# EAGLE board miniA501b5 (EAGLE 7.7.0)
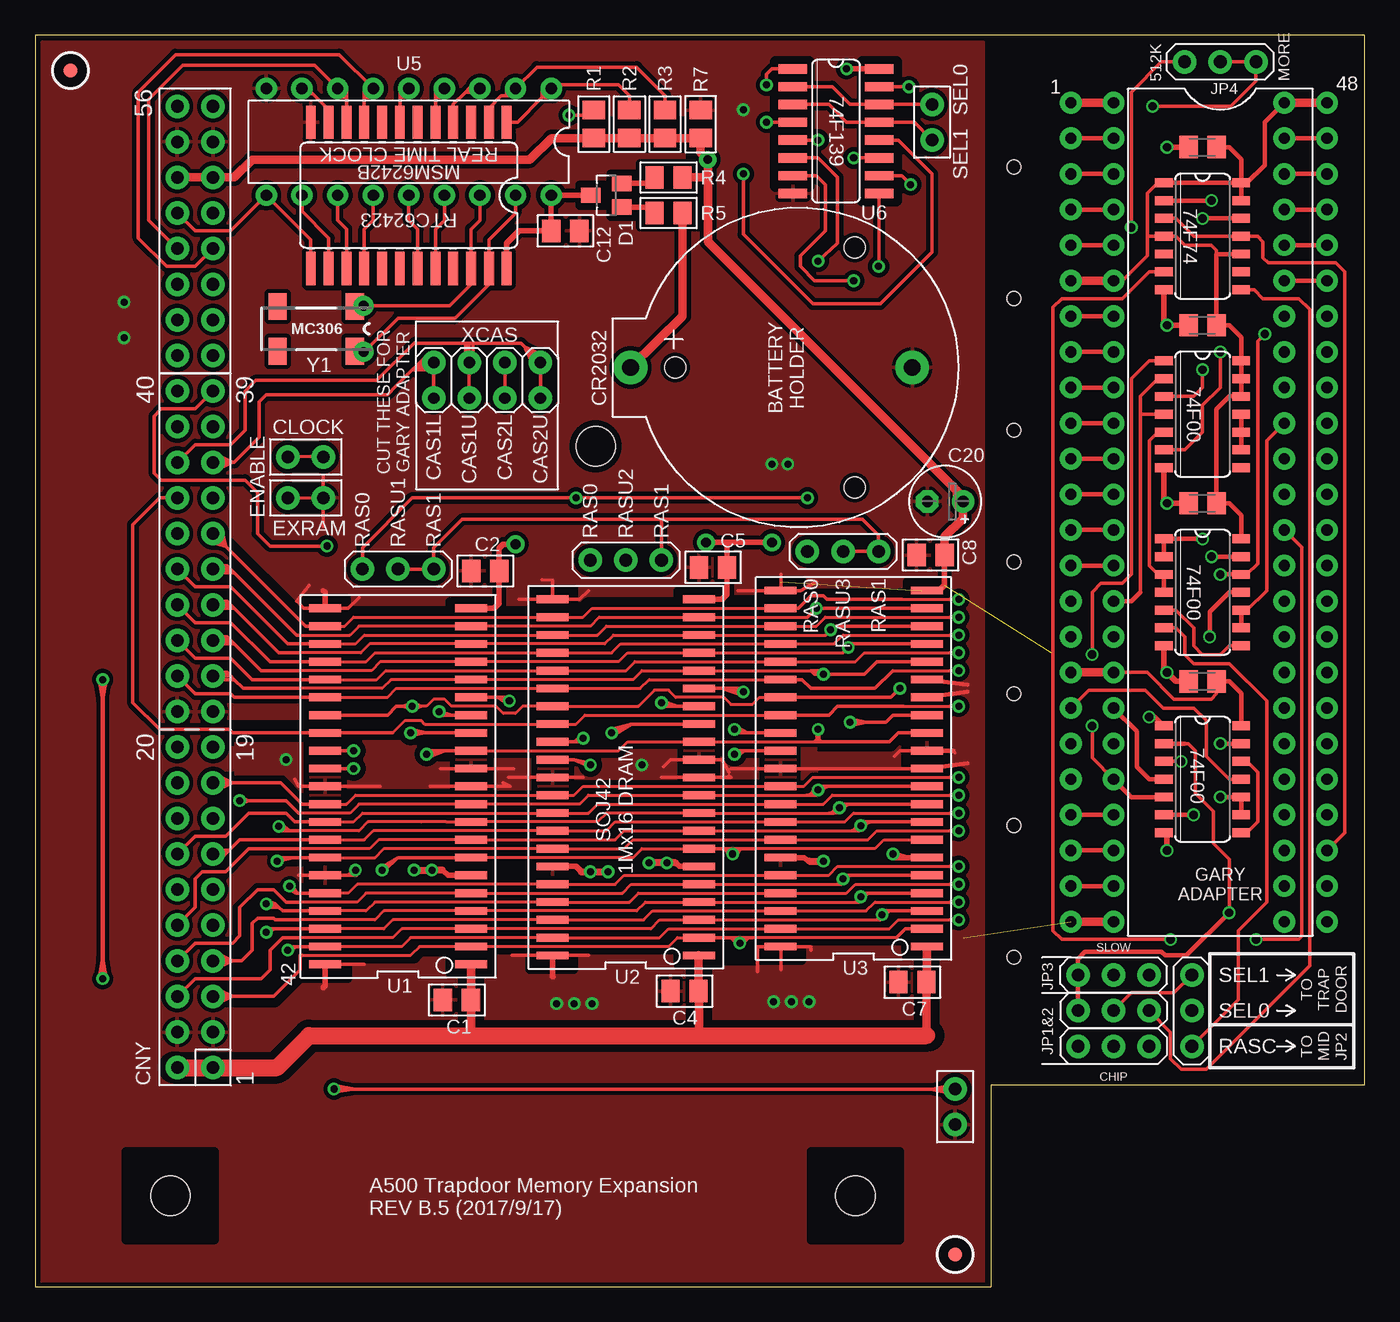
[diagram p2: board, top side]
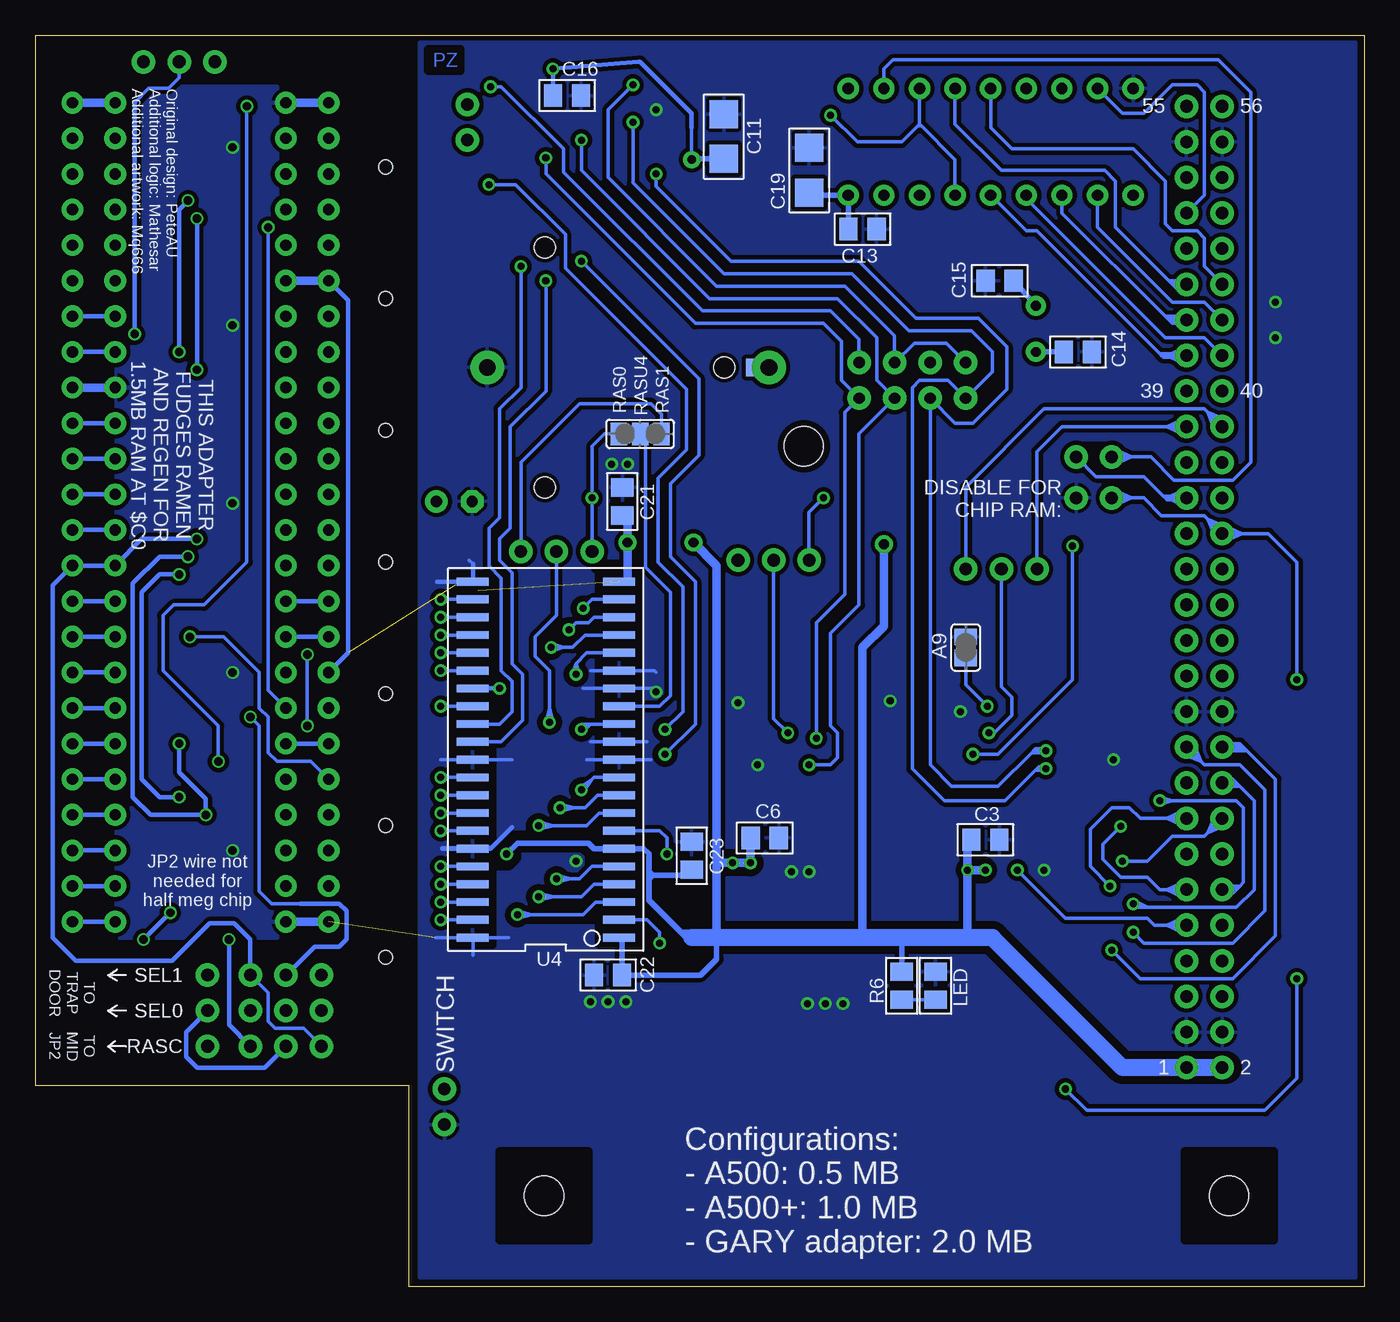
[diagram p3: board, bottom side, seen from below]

Size 94.87 x 89.28 mm. Coordinates in mm from the lower left corner, seen from the top.
Outline: 0,0 68.2,0 68.2,14.35 94.87,14.35 94.87,89.28 0,89.28 0,0
Copper layers (1*16): Top 0.035mm / dielectric 1.5mm / Bottom 0.035mm
Design rules "SeeedStudio_DRU_no_angle_2layer *": minimum track width 6mil, minimum drill 12mil, track to track 10mil, track to pad 10mil, pad to pad 10mil, via to via 10mil, smd to smd 0mil, copper to edge 10mil, drill to drill 10mil, minimum pad ring 10mil, minimum via ring 6mil, stop-mask expansion 2mil, vias tented up to drill 25mil, thermal gap 10mil
Holes 2.8 mm at 9.65,6.48 58.55,6.48 40.01,59.94
Holes 1 mm at 69.85,51.69 69.85,32.89 69.85,70.48 69.85,79.88 69.85,42.29 69.85,23.49 69.85,61.09
tRestrict: area 19.2,22 to 22.4,23.5; area 19.2,47.6 to 22.2,49.1; area 45.8,34.7 to 46,43.2; area 45.8,35.3 to 46,38.1; area 38.4,34.7 to 38.5,38; area 22.1,34.9 to 22.2,36.7; area 35.4,47.4 to 38.5,49.8; area 32.6,41.1 to 34.7,42.4; area 27.9,40.4 to 29.7,41.7; area 38.4,28.8 to 42.9,30.4; area 54.6,28.6 to 58.3,31.2; area 48.9,41.9 to 50.9,43.2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; 65 lines
bRestrict: area 64.5,86.7 to 66.8,88.3; area 6.5,3.3 to 12.8,9.7; area 55.4,3.3 to 61.7,9.7; area 52.8,42.8 to 53.6,43.8; area 52.8,37.7 to 53.6,38.7; area 62.2,49.9 to 65.2,50.8; area 51.8,50.7 to 54.5,50.8; area 62.2,24.4 to 64.8,24.5; area 55.4,39.3 to 56.3,40.2; area 55.8,43.2 to 56.7,44.1; area 55.3,47.9 to 56.2,48.8; area 56.3,46.4 to 57.2,47.3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; 15 lines

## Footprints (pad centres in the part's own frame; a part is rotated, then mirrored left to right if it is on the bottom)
SJ = smd 1.168 x 1.6: 1 -0.762,0; 2 0.762,0
CR2032-THRU = drill 1.2 pad 2.4: + 0,-11.1; - 0,9 | smd 1.27 x 0.635 bottom: +2 0,-9.763 | hole 1.5: 8.55,4.9; 0,-7.9; -8.55,4.9
C0805KPZ = smd 1.3 x 1.6: P$1 -1,0; P$2 1,0
C0805K = smd 1.3 x 1.6: 1 -1,0; 2 1,0
C1206PZ = smd 2 x 2.05: P$1 -1.6,0; P$2 1.6,0
E2,5-5 = drill 0.813 pad 1.6: + -1.27,0 | drill 0.813 pad 1.6 octagon: - 1.27,0
1X02 = drill 0.9 pad 1.676: 1 -1.27,0; 2 1.27,0
2X20 = drill 0.9 pad 1.676: 1 -24.13,-1.27; 2 -24.13,1.27; 3 -21.59,-1.27; 4 -21.59,1.27; 5 -19.05,-1.27; 6 -19.05,1.27; 7 -16.51,-1.27; 8 -16.51,1.27; 9 -13.97,-1.27; 10 -13.97,1.27; 11 -11.43,-1.27; 12 -11.43,1.27; 13 -8.89,-1.27; 14 -8.89,1.27; 15 -6.35,-1.27; 16 -6.35,1.27; 17 -3.81,-1.27; 18 -3.81,1.27; 19 -1.27,-1.27; 20 -1.27,1.27; 21 1.27,-1.27; 22 1.27,1.27; 23 3.81,-1.27; 24 3.81,1.27; 25 6.35,-1.27; 26 6.35,1.27; 27 8.89,-1.27; 28 8.89,1.27; 29 11.43,-1.27; 30 11.43,1.27; 31 13.97,-1.27; 32 13.97,1.27; 33 16.51,-1.27; 34 16.51,1.27; 35 19.05,-1.27; 36 19.05,1.27; 37 21.59,-1.27; 38 21.59,1.27; 39 24.13,-1.27; 40 24.13,1.27
2X08 = drill 0.9 pad 1.676: 1 -8.89,-1.27; 2 -8.89,1.27; 3 -6.35,-1.27; 4 -6.35,1.27; 5 -3.81,-1.27; 6 -3.81,1.27; 7 -1.27,-1.27; 8 -1.27,1.27; 9 1.27,-1.27; 10 1.27,1.27; 11 3.81,-1.27; 12 3.81,1.27; 13 6.35,-1.27; 14 6.35,1.27; 15 8.89,-1.27; 16 8.89,1.27
SOT23 = smd 1.1 x 1.4: 1 -0.85,-1.1; 2 0.85,-1.1; 3 0,1.1
DIL48 = drill 0.8 pad 1.55: 1 -29.21,-7.62; 2 -26.67,-7.62; 3 -24.13,-7.62; 4 -21.59,-7.62; 5 -19.05,-7.62; 6 -16.51,-7.62; 7 -13.97,-7.62; 8 -11.43,-7.62; 9 -8.89,-7.62; 10 -6.35,-7.62; 11 -3.81,-7.62; 12 -1.27,-7.62; 13 1.27,-7.62; 14 3.81,-7.62; 15 6.35,-7.62; 16 8.89,-7.62; 17 11.43,-7.62; 18 13.97,-7.62; 19 16.51,-7.62; 20 19.05,-7.62; 21 21.59,-7.62; 22 24.13,-7.62; 23 26.67,-7.62; 24 29.21,-7.62; 25 29.21,7.62; 26 26.67,7.62; 27 24.13,7.62; 28 21.59,7.62; 29 19.05,7.62; 30 16.51,7.62; 31 13.97,7.62; 32 11.43,7.62; 33 8.89,7.62; 34 6.35,7.62; 35 3.81,7.62; 36 1.27,7.62; 37 -1.27,7.62; 38 -3.81,7.62; 39 -6.35,7.62; 40 -8.89,7.62; 41 -11.43,7.62; 42 -13.97,7.62; 43 -16.51,7.62; 44 -19.05,7.62; 45 -21.59,7.62; 46 -24.13,7.62; 47 -26.67,7.62; 48 -29.21,7.62
SO14 = smd 0.635 x 1.27: 1 -3.81,-2.756; 2 -2.54,-2.756; 3 -1.27,-2.756; 4 0,-2.756; 5 1.27,-2.756; 6 2.54,-2.756; 7 3.81,-2.756; 8 3.81,2.756; 9 2.54,2.756; 10 1.27,2.756; 11 0,2.756; 12 -1.27,2.756; 13 -2.54,2.756; 14 -3.81,2.756
1X03 = drill 0.9 pad 1.676: 1 -2.54,0; 2 0,0; 3 2.54,0
1X01 = drill 0.7 pad 1.422: 1 0,0
2X04 = drill 0.813 pad 1.676: 1 -3.81,-1.27; 2 -3.81,1.27; 3 -1.27,-1.27; 4 -1.27,1.27; 5 1.27,-1.27; 6 1.27,1.27; 7 3.81,-1.27; 8 3.81,1.27
M0805PZ = smd 1.3 x 1.6: P$1 -1,0; P$2 1,0
SJ_2 = smd 1.168 x 1.6: 1 -1.524,0; 2 0,0; 3 1.524,0
SOJ40 = smd 0.559 x 2.286: 1 -10.16,-5.22; 2 -8.89,-5.22; 3 -7.62,-5.22; 4 -6.35,-5.22; 5 -5.08,-5.22; 6 -3.81,-5.22; 7 -2.54,-5.22; 8 -1.27,-5.22; 9 0,-5.22; 10 1.27,-5.22; 11 2.54,-5.22; 12 3.81,-5.22; 13 5.08,-5.22; 14 6.35,-5.22; 15 7.62,-5.22; 16 8.89,-5.22; 17 10.16,-5.22; 18 11.43,-5.22; 19 12.7,-5.22; 20 13.97,-5.22; 21 15.24,-5.22; 22 15.24,5.22; 23 13.97,5.22; 24 12.7,5.22; 25 11.43,5.22; 26 10.16,5.22; 27 8.89,5.22; 28 7.62,5.22; 29 6.35,5.22; 30 5.08,5.22; 31 3.81,5.22; 32 2.54,5.22; 33 1.27,5.22; 34 0,5.22; 35 -1.27,5.22; 36 -2.54,5.22; 37 -3.81,5.22; 38 -5.08,5.22; 39 -6.35,5.22; 40 -7.62,5.22; 41 -8.89,5.22; 42 -10.16,5.22
DIL18 = drill 0.813 pad 1.524: 1 -10.16,-3.81; 2 -7.62,-3.81; 3 -5.08,-3.81; 4 -2.54,-3.81; 5 0,-3.81; 6 2.54,-3.81; 7 5.08,-3.81; 8 7.62,-3.81; 9 10.16,-3.81; 10 10.16,3.81; 11 7.62,3.81; 12 5.08,3.81; 13 2.54,3.81; 14 0,3.81; 15 -2.54,3.81; 16 -5.08,3.81; 17 -7.62,3.81; 18 -10.16,3.81
SO16 = smd 0.66 x 2.032: 1 -4.445,-3.073; 2 -3.175,-3.073; 3 -1.905,-3.073; 4 -0.635,-3.073; 5 0.635,-3.073; 6 1.905,-3.073; 7 3.175,-3.073; 8 4.445,-3.073; 9 4.445,3.073; 10 3.175,3.073; 11 1.905,3.073; 12 0.635,3.073; 13 -0.635,3.073; 14 -1.905,3.073; 15 -3.175,3.073; 16 -4.445,3.073
SOP24 = smd 0.711 x 2.362: 1 -6.985,-5.22; 2 -5.715,-5.22; 3 -4.445,-5.22; 4 -3.175,-5.22; 5 -1.905,-5.22; 6 -0.635,-5.22; 7 0.635,-5.22; 8 1.905,-5.22; 9 3.175,-5.22; 10 4.445,-5.22; 11 5.715,-5.22; 12 6.985,-5.22; 13 6.985,5.22; 14 5.715,5.22; 15 4.445,5.22; 16 3.175,5.22; 17 1.905,5.22; 18 0.635,5.22; 19 -0.635,5.22; 20 -1.905,5.22; 21 -3.175,5.22; 22 -4.445,5.22; 23 -5.715,5.22; 24 -6.985,5.22
FIDUCIAL_1MM = smd 1 x 1: 1 0,0
MC-306 = smd 1.3 x 1.9: 1 -2.75,-1.6; 2 2.75,-1.6; 3 2.75,1.6; 4 -2.75,1.6

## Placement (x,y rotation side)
A9  [SJ]  28.45,45.59 270 bottom
BAT1  [CR2032-THRU]  53.59,65.57 270 top
C1  100nF  [C0805KPZ]  30.1,20.45 0 top
C2  100nF  [C0805KPZ]  32.13,51.05 0 top
C3  100nF  [C0805KPZ]  27.05,31.88 180 bottom
C4  100nF  [C0805KPZ]  46.35,21.08 0 top
C5  100nF  [C0805KPZ]  48.39,51.31 0 top
C6  100nF  [C0805KPZ]  42.8,32 180 bottom
C7  100nF  [C0805KPZ]  62.61,21.72 0 top
C8  100nF  [C0805KPZ]  63.91,52.19 0 top
C9  100n  [C0805K]  83.31,43.18 180 top
C11  TANT  [C1206PZ]  45.72,82.04 90 bottom
C12  100nF  [C0805KPZ]  37.85,75.31 180 top
C13  4.7uF 10V  [C0805KPZ]  35.81,75.44 0 bottom
C14  22pF  [C0805KPZ]  20.45,66.67 0 bottom
C15  22pF  [C0805KPZ]  26.04,71.75 180 bottom
C16  100nF  [C0805KPZ]  56.9,84.96 0 bottom
C17  100n  [C0805K]  83.31,55.88 180 top
C18  100n  [C0805K]  83.31,68.58 180 top
C19  [C1206PZ]  39.62,79.63 90 bottom
C20  [E2,5-5]  64.95,56.01 180 top
C21  100nF  [C0805KPZ]  52.96,56.01 270 bottom
C22  100nF  [C0805KPZ]  53.98,22.23 0 bottom
C23  100nF  [C0805KPZ]  48.01,30.73 270 bottom
C24  100n  [C0805K]  83.31,81.28 180 top
CLOCK  [1X02]  19.3,59.18 0 top
CNY  [2X20]  11.43,39.75 90 top
CNY2  [2X08]  11.43,75.31 90 top
D1  BAT721C  [SOT23]  40.77,77.85 90 top
EXRAM  [1X02]  19.3,56.26 0 top
GARY  [DIL48]  84.58,55.24 270 top
IC1  74F00  [SO14]  83.31,36.2 270 top
IC2  74F00  [SO14]  83.31,49.53 270 top
IC3  74F00  [SO14]  83.31,62.23 270 top
IC4  74F74  [SO14]  83.31,74.93 270 top
J8  [1X03]  82.55,19.68 90 top
JP1  [1X03]  25.91,51.18 0 top
JP2  [1X03]  76.96,17.14 0 top
JP3  [1X01]  23.44,66.67 0 top
JP4  [1X01]  23.44,69.98 0 top
JP5  [1X03]  57.66,52.45 0 top
JP6  [1X03]  76.96,19.68 0 top
JP7  [1X03]  42.16,51.82 0 top
JP8  [1X03]  76.96,22.23 180 top
JP9  [1X03]  84.58,87.38 180 top
JP10  [2X04]  32.26,64.64 180 top
LED  LED  [M0805PZ]  30.61,21.46 270 bottom
R1  10K  [M0805PZ]  39.88,82.93 270 top
R2  10K  [M0805PZ]  42.42,82.93 270 top
R3  10K  [M0805PZ]  44.96,82.93 270 top
R4  470  [M0805PZ]  45.21,79.12 0 top
R5  470  [M0805PZ]  45.21,76.58 0 top
R6  1K  [M0805PZ]  33.02,21.46 90 bottom
R7  100K  [C0805KPZ]  47.5,82.93 90 top
SEL[0_1]  [1X02]  64.01,83.06 270 top
SJ1  [SJ_2]  51.69,60.83 0 bottom
SOCKET(MOBO)  [DIL48]  81.53,55.24 270 top
SWITCH  [1X02]  65.66,12.83 270 top
U1  [SOJ40]  25.91,33.15 90 top
U2  [SOJ40]  42.16,33.78 90 top
U3  [SOJ40]  58.42,34.42 90 top
U4  [SOJ40]  58.42,35.05 90 bottom
U5  OKI MSM6242B  [DIL18]  26.67,81.66 180 top
U6  74F139D  [SO16]  57.15,82.42 270 top
U55  RTC72421SOP24  [SOP24]  26.67,77.85 180 top
U$1  FIDUCIAL  [FIDUCIAL_1MM]  2.54,86.74 0 top
U$2  FIDUCIAL  [FIDUCIAL_1MM]  65.66,2.29 0 top
Y1  MC-306  [MC-306]  20.07,68.33 180 top

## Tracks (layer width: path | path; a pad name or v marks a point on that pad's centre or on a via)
/A19
  Top 0.254: 80.14,50.8 79.5,51.43 79.5,60.32 80.14,60.96
  Top 0.305: IC2.4 IC2.3 80.14,50.8 | 80.14,60.96 IC3.5
/A19_FF  (via drill 0.6)
  Top 0.254: v81.03,24.77 73.28,24.77 72.64,25.4 72.64,69.85 73.28,70.48 77.6,70.48 79.5,72.39 IC4.6
  Bottom 0.305: JP2.3 81.03,18.67 v81.03,24.77
/BLIT
  Top 0.254: 78.87,49.53 78.87,62.23 | 78.87,62.23 78.87,63.5 80.14,64.77 | IC3.4 78.87,62.23
  Top 0.305: GARY.15 78.23,48.89 78.87,49.53 | 80.14,64.77 IC3.2
  Bottom 0.305: SOCKET(MOBO).15 GARY.15
/GARY_RAMEN  (via drill 0.6)
  Top 0.254: GARY.20 75.44,37.72 v75.44,40 | v75.44,45.09 75.44,49.53 76.07,50.16 77.6,50.16 78.23,50.8 78.23,64.77 79.5,66.04 IC3.1
  Top 0.305: IC1.5 78.23,34.92 GARY.20
  Bottom 0.254: v75.44,40 v75.44,45.09
/GARY_RAMEN_FF
  Top 0.254: IC4.8 87,71.12 87.63,70.48 90.2,70.48 90.96,69.72 90.96,22.88 83.57,15.49 81.79,15.49 81.03,16.26 81.03,18.16 JP6.3
/GARY_REGEN  (via drill 0.6)
  Top 0.254: v78.23,75.56 78.23,85.22 80.39,87.38 JP9.3
  Top 0.305: IC1.4 79.5,36.2 78.61,37.08 78.61,39.62 GARY.18
  Bottom 0.254: GARY.18 78.23,42.54 v78.23,75.56
/NEW_RAMEN  (via drill 0.6)
  Top 0.305: IC2.11 85.22,49.53 83.82,48.13 v83.82,46.35
  Bottom 0.254: SOCKET(MOBO).20 75.18,37.46 77.6,37.46 78.23,38.1 78.23,40.64 78.87,41.27 78.87,43.81 81.41,46.35 v83.82,46.35
/NEW_REGEN
  Top 0.254: IC1.11 85.22,36.2 83.57,37.85 83.57,40.39 82.68,41.27 80.52,41.27 79.25,42.54 75.18,42.54 SOCKET(MOBO).18
A0  (via drill 0.5 pad 0.9)
  Top 0.203: 18.8,42.67 24.77,42.67 25.4,43.31 U1.17 42.67,43.31 43.31,43.94 U2.17 55.37,43.94
  Top 0.254: U3.17 60.07,44.58 59.18,43.69 v56.26,43.69 55.63,43.69 55.37,43.94 56.26,43.94 | CNY.23 13.97,43.56 | 13.97,43.56 14.22,43.31 | 14.22,43.31 14.86,42.67 18.8,42.67 | 14.22,43.31 12.7,43.31 | 13.97,43.56 13.72,43.81 12.7,43.81
  Bottom 0.254: U4.17 55.5,45.21 56.26,44.45 | 56.26,44.45 v56.26,43.69 | 56.26,44.45 56.01,43.69 | 56.26,44.45 56.52,43.69
A1  (via drill 0.5 pad 0.9)
  Top 0.203: 18.8,43.94 24,43.94 24.64,44.58 U1.18 41.66,44.58 42.29,45.21 U2.18 57.66,45.21
  Top 0.254: 18.8,43.94 16.13,43.94 14.22,45.85 | 57.66,45.21 v58.04,45.59 58.29,45.85 U3.18 | 14.22,45.85 13.97,46.1 | 13.97,46.1 CNY.25 | 14.22,45.85 12.7,45.85 | 13.97,46.1 13.72,46.35 12.7,46.35
  Bottom 0.254: U4.18 55.63,46.48 56.52,45.59 57.15,45.59 | 57.15,45.59 v58.04,45.59 | 57.15,45.59 58.04,45.85 | 57.15,45.59 58.04,45.34
A2  (via drill 0.5 pad 0.9)
  Top 0.203: 18.8,45.21 23.24,45.21 23.88,45.85 U1.19 40.64,45.85 41.27,46.48 U2.19 56.39,46.48
  Top 0.254: 18.8,45.21 17.4,45.21 14.22,48.39 | 56.39,46.48 v56.77,46.86 57.02,47.12 U3.19 | CNY.27 13.97,48.64 | 13.97,48.64 14.22,48.39 | 14.22,48.39 12.7,48.39 | 13.97,48.64 13.72,48.89 12.7,48.89
  Bottom 0.254: U4.19 54.99,47.75 55.37,47.37 56.26,47.37 v56.77,46.86
A3  (via drill 0.5 pad 0.9)
  Top 0.203: 55.12,47.75 U2.20 40.26,47.75 39.62,47.12 U1.20 23.11,47.12 22.48,46.48 18.8,46.48
  Top 0.254: 55.12,47.75 v55.75,48.39 U3.20 | 18.8,46.48 18.67,46.48 14.22,50.93 | CNY.29 13.97,51.18 | 13.97,51.18 14.22,50.93 | 14.22,50.93 12.7,50.93 | 13.97,51.18 13.72,51.43 12.7,51.43
  Bottom 0.254: U4.20 55.12,49.02 v55.75,48.39
A4  (via drill 0.5 pad 0.9)
  Top 0.203: U1.23 22.1,47.12 22.73,47.75 U2.23 39.12,47.75 39.75,48.39 U3.23 | 61.85,49.02 65.28,49.02
  Top 0.254: U1.23 19.3,47.12 13.59,52.83 | U3.23 54.48,48.39 55.37,49.28 56.26,49.28 56.52,49.02 61.85,49.02 | 65.28,49.02 v65.91,49.02 | CNY.31 13.59,52.83 | 13.59,52.83 12.57,53.09 | 13.59,52.83 13.34,53.97
  Bottom 0.254: v65.91,49.02 U4.23
A5  (via drill 0.5 pad 0.9)
  Top 0.203: U1.24 22.86,45.85 23.49,46.48 U2.24 | 36.96,46.48 U2.24 | U2.24 40.13,46.48 40.77,47.12 U3.24 55.75,47.12 56.39,47.75 65.28,47.75
  Top 0.254: U1.24 18.03,45.85 13.97,49.91 11.43,49.91 CNY.30 | 65.28,47.75 v65.91,47.75
  Bottom 0.254: v65.91,47.75 U4.24
A6  (via drill 0.5 pad 0.9)
  Top 0.203: U1.25 23.62,44.58 24.26,45.21 U2.25 | 36.96,45.21 U2.25 | U2.25 41.15,45.21 41.78,45.85 U3.25 57.02,45.85 57.66,46.48 65.28,46.48
  Top 0.254: U1.25 16.76,44.58 13.97,47.37 11.43,47.37 CNY.28 | 65.28,46.48 v65.91,46.48
  Bottom 0.254: v65.91,46.48 U4.25
A7  (via drill 0.5 pad 0.9)
  Top 0.203: U1.26 24.38,43.31 25.02,43.94 U2.26 42.16,43.94 42.8,44.58 U3.26 58.55,44.58 59.18,45.21 65.28,45.21
  Top 0.254: U1.26 15.49,43.31 13.97,44.83 11.43,44.83 CNY.26 | 65.28,45.21 v65.91,45.21
  Bottom 0.254: v65.91,45.21 U4.26
A8  (via drill 0.5 pad 0.9)
  Top 0.203: U1.27 25.15,42.04 25.78,42.67 U2.27 43.18,42.67 43.81,43.31 U3.27 | 61.21,43.94 65.28,43.94
  Top 0.254: 61.21,43.94 59.94,42.67 55.37,42.67 54.74,43.31 U3.27 | 65.28,43.94 v65.91,43.94 | CNY.24 11.43,42.29 13.97,42.29 14.22,42.04 U1.27
  Bottom 0.254: U4.27 v65.91,43.94
A9  (via drill 0.5 pad 0.9)
  Top 0.203: 27.56,41.4 27.94,41.4 28.45,41.91 29.21,41.91 29.72,41.4 32.89,41.4 33.4,40.89 34.29,40.89 34.8,41.4 U2.28 43.05,41.4 44.2,42.54 45.21,42.54 45.72,42.04 49.15,42.04 49.66,41.53 51.18,41.53 51.69,42.04 U3.28 | 27.56,41.4 v26.92,41.4 | 26.92,41.15 27.56,41.4 | 27.56,41.4 26.92,41.66
  Top 0.254: 26.29,41.4 25.78,41.4 25.15,40.77 U1.28 | 26.29,41.4 v26.92,41.4 | 26.29,41.4 26.92,41.15 | 26.29,41.4 26.92,41.66 | v61.72,42.67 61.09,42.04 U3.28
  Bottom 0.254: 28.45,46.1 A9.2 28.45,42.93 v26.92,41.4
  Bottom 0.305: v61.72,42.67 U4.28
A19
  Top 0.254: U6.2 56.9,85.6 58.17,84.33 U6.14 SEL[0_1].1
A20
  Top 0.254: U6.3 56.64,84.33 57.91,83.06 U6.13 62.74,83.06 SEL[0_1].2
A23
  Top 0.254: SOCKET(MOBO).39 87.88,60.32 87.88,49.66 86.49,48.26
  Top 0.305: 86.49,48.26 IC2.10 IC2.9
  Bottom 0.305: GARY.39 SOCKET(MOBO).39
ALE  (via drill 0.5 pad 0.9)
  Top 0.254: 40.13,83.44 R1.P$1 39.51,83.57 v38.1,83.57 | U55.20 28.57,75.44 29.21,76.07 U5.15 | U55.4 29.84,84.33 30.73,85.22 | 30.73,85.22 30.99,85.47 U5.3 | 30.73,85.22 31.88,85.22
  Bottom 0.254: U5.3 31.75,82.93 | 31.75,82.93 31.62,82.8 | 31.62,82.8 29.21,80.39 U5.15 | v38.1,83.57 36.2,81.66 33.02,81.66 31.88,82.8 | 31.88,82.8 31.75,82.93 | 31.62,82.8 31.88,82.8
CASL_U1  (via drill 0.5 pad 0.9)
  Top 0.203: 22.61,37.21 22.22,36.96 22.61,36.7
  Top 0.254: U1.31 22.22,36.96 v22.73,36.96 | U6.4 v52.2,83.06
  Bottom 0.254: v22.73,36.96 23.37,36.96 | 23.37,36.96 23.49,36.83 | 23.49,36.83 25.65,34.67 29.97,34.67 32.26,36.96 32.26,64.14 31.75,64.64 29.72,64.64 JP10.8 26.54,65.28 26.54,66.67 28.07,68.2 32.51,68.2 36.58,72.26 45.72,72.26 52.2,78.74 v52.2,83.06 | 23.49,36.83 22.73,36.83 | 23.37,36.96 23.24,37.08 22.73,37.08
CASL_U2  (via drill 0.5 pad 0.9)
  Top 0.254: U2.31 38.48,37.59 | 38.48,37.59 v39.62,37.21 | v55.88,81.79 U6.5 | 38.48,37.59 39.62,37.08 | 38.48,37.59 39.62,37.34
  Bottom 0.254: v55.88,81.79 55.88,79.63 46.74,70.48 37.59,70.48 34.8,67.69 34.8,64.64 JP10.4 36.07,60.83 36.07,48.64 38.1,46.61 38.1,40 37.59,39.5 37.59,37.72 38.1,37.21 v39.62,37.21
CASL_U3  (via drill 0.5 pad 0.9)
  Top 0.254: U6.6 55.88,80.52 57.28,79.12 57.28,74.42 v55.88,73.15 | U3.31 50.67,38.23 | 50.67,38.23 v49.91,37.97 | 50.67,38.23 49.91,37.72 | 50.67,38.23 49.91,38.23
  Bottom 0.254: v49.91,37.97 47.75,40.13 47.75,50.29 49.53,52.07 49.53,57.28 47.5,59.31 47.5,64.77 v55.88,73.15
CASL_U4  (via drill 0.5 pad 0.9)
  Top 0.254: U6.7 55.75,79.25 56.39,78.61 56.39,75.31 54.61,73.53 54.61,72.77 55.63,71.75 v58.42,71.75
  Bottom 0.254: U4.31 61.59,38.86 60.07,40.39 60.07,43.69 60.83,44.45 60.83,50.93 61.72,51.82 61.72,53.34 60.96,54.1 60.96,61.34 58.42,63.88 v58.42,71.75
CASU_U1  (via drill 0.5 pad 0.9)
  Top 0.203: 22.61,38.48 22.22,38.23 22.61,37.97
  Top 0.254: v22.73,38.23 22.22,38.23 U1.30 | v50.55,79.38 50.55,75.06 55.5,70.1 60.32,70.1 64.01,73.79 64.01,79.38 61.59,81.79 U6.12
  Bottom 0.254: v22.73,38.23 23.62,38.23 | 23.62,38.23 23.75,38.1 | 23.75,38.1 26.16,35.69 29.46,35.69 30.99,37.21 JP10.6 29.21,61.59 27.94,61.59 25.53,64.01 25.53,67.06 27.56,69.09 32,69.09 36.07,73.15 45.21,73.15 50.55,78.49 v50.55,79.38 | 22.73,38.1 23.75,38.1 | 23.62,38.23 23.49,38.35 22.73,38.35
CASU_U2  (via drill 0.5 pad 0.9)
  Top 0.254: U2.30 38.48,38.86 | 38.48,38.86 v39.12,39.12 | U6.11 v58.42,80.52 | 38.48,38.86 39.12,38.86 | 38.48,38.86 39.12,39.37
  Bottom 0.254: v39.12,39.12 39.12,47.37 37.08,49.4 37.08,62.36 JP10.2 37.34,64.64 37.34,67.44 38.61,68.71 47.75,68.71 58.42,79.38 v58.42,80.52
CASU_U3  (via drill 0.5 pad 0.9)
  Top 0.254: U3.30 50.8,39.5 | 50.8,39.5 v49.91,39.75 | U6.10 61.85,79.25 v62.48,78.61 | 50.8,39.5 49.91,39.5 | 50.8,39.5 49.91,40
  Bottom 0.254: v49.91,39.75 48.64,41.02 48.64,49.91 50.42,51.69 50.42,57.66 48.39,59.69 48.39,64.01 57.02,72.64 57.02,75.06 60.58,78.61 v62.48,78.61
CASU_U4  (via drill 0.5 pad 0.9)
  Top 0.254: U6.9 60.22,72.8 v60.2,72.77
  Bottom 0.254: U4.30 61.72,40.13 60.83,41.02 60.83,43.18 61.59,43.94 61.59,50.55 62.48,51.43 62.48,54.1 61.72,54.86 61.72,62.61 60.2,64.14 v60.2,72.77
CCKQ
  Top 0.254: IC4.3 81.41,76.2 82.68,74.93 IC4.11 87.25,74.93 87.63,74.55 87.63,73.41 88.01,73.03 92.84,73.03 93.47,72.39 93.47,32.38 GARY.27
  Bottom 0.305: SOCKET(MOBO).27 GARY.27
CS0
  Top 0.254: R3.P$1 44.96,84.96 42.93,87 35.81,87 U5.2 34.04,85.47 33.53,84.96 | 33.53,84.96 33.66,84.96 | 33.66,84.96 34.29,84.96 | 33.66,84.96 33.66,85.47 | U55.2 32.38,84.07 33.27,84.96 33.53,84.96
  Bottom 0.254: U5.2 34.29,86.87 33.66,87.5 10.41,87.5 8.13,85.22 8.13,58.8 9.4,57.53 13.59,57.53 15.24,59.18 16.64,59.18 | CLOCK.1 16.64,59.18 | 16.64,59.18 18.03,58.55 | 16.64,59.18 18.03,59.82
D0  (via drill 0.5 pad 0.9)
  Top 0.203: U2.2 45.85,24.89 45.21,24.26 U1.2 27.43,24.26 26.8,23.62 19.05,23.62 | 61.47,24.89 51.18,24.89 | 50.42,24.38 v50.29,24.51
  Top 0.254: 14.1,20.7 17.02,20.7 18.92,22.61 18.92,23.62 19.05,23.62 | 14.1,20.7 CNY.5 | U2.2 49.66,24.89 | 49.66,24.89 50.29,24.89 | U3.2 62.1,25.53 61.47,24.89 | v50.29,24.51 50.29,24.89 | 49.66,24.89 50.16,24.38 | 50.93,24.89 50.42,24.38 | 50.29,24.89 50.93,24.89 | 50.93,24.89 51.18,24.89 | 14.1,20.7 12.7,20.07 | 14.1,20.7 12.7,21.34
  Bottom 0.254: v50.29,24.51 50.29,25.27 51.18,26.16 U4.2
D1  (via drill 0.5 pad 0.9)
  Top 0.203: 18.8,24.89 25.53,24.89 26.16,25.53 U1.3 43.94,25.53 44.58,26.16 U2.3 60.07,26.16
  Top 0.254: CNY.6 11.43,21.97 16.13,21.97 16.76,22.61 16.76,24 17.65,24.89 18.8,24.89 | 60.96,26.8 60.71,26.8 v60.45,26.54 60.07,26.16 60.32,26.16 60.96,26.8 | 60.96,26.8 U3.3
  Bottom 0.254: U4.3 54.86,27.43 55.75,26.54 59.44,26.54 | 59.44,26.54 v60.45,26.54 | 59.44,26.54 60.45,26.8 | 59.44,26.54 60.45,26.29
D2  (via drill 0.5 pad 0.9)
  Top 0.203: 18.8,26.16 24.26,26.16 24.89,26.8 U1.4 42.93,26.8 43.56,27.43 U2.4 58.55,27.43
  Top 0.254: 18.8,26.16 17.14,26.16 17.02,26.29 15.88,26.29 15.49,25.91 15.49,24 14.73,23.24 14.1,23.24 | 14.1,23.24 CNY.7 | 59.44,28.07 59.18,28.07 v58.93,27.81 58.55,27.43 58.8,27.43 59.44,28.07 | 59.44,28.07 U3.4 | 14.1,23.24 12.7,23.88 | 14.1,23.24 12.7,22.61
  Bottom 0.254: U4.4 54.99,28.7 55.88,27.81 57.91,27.81 | 57.91,27.81 v58.93,27.81 | 57.91,27.81 58.93,28.07 | 57.91,27.81 58.93,27.56
D3  (via drill 0.5 pad 0.9)
  Top 0.203: 18.8,27.43 22.99,27.43 23.62,28.07 U1.5 41.91,28.07 42.55,28.7 U2.5 57.28,28.7
  Top 0.254: CNY.8 11.43,24.51 14.1,24.51 14.61,25.02 14.61,27.05 15.88,28.32 17.02,28.32 17.91,27.43 18.8,27.43 | 58.17,29.34 57.91,29.34 v57.66,29.08 57.28,28.7 57.53,28.7 58.17,29.34 | 58.17,29.34 U3.5
  Bottom 0.254: U4.5 55.12,29.97 56.01,29.08 56.64,29.08 | 56.64,29.08 v57.66,29.08 | 56.64,29.08 57.66,28.83 | 56.64,29.08 57.66,29.34
D4  (via drill 0.5 pad 0.9)
  Top 0.203: U1.7 42.67,30.61 43.31,31.24 U2.7 | U3.7 60.58,31.88 59.94,31.24 51.31,31.24 | 24.64,29.84 25.91,30.61 24.89,29.59
  Top 0.254: U1.7 25.91,30.61 v24.77,29.72 | U2.7 49.28,31.24 | 49.28,31.24 49.78,31.24 | 51.31,31.24 50.29,31.24 | 50.29,31.24 49.78,31.24 | 49.78,31.24 v49.78,30.86 | v49.78,30.86 49.91,30.61 50.29,31.24 | v49.78,30.86 49.66,30.61 49.28,31.24
  Bottom 0.254: CNY.9 14.1,25.78 | 14.1,25.78 14.99,25.78 15.49,26.29 21.34,26.29 v24.77,29.72 | U4.7 50.29,32.51 49.78,32 v49.78,30.86 | 14.1,25.78 12.7,25.15 | 14.1,25.78 12.7,26.42
D5  (via drill 0.5 pad 0.9)
  Top 0.203: 18.8,31.24 23.88,31.24 24.51,31.88 U1.8 41.4,31.88 42.04,32.51 U2.8 58.19,32.51 | 58.19,32.51 58.52,32.51 | 58.52,32.51 58.55,32.51 v58.93,32.89 | 58.52,32.51 arc11 59.05,32.56 | 58.19,32.51 arc93 58.6,32.94
  Top 0.254: 18.8,31.24 15.24,31.24 13.59,29.59 11.94,29.59 11.43,29.08 11.43,27.05 CNY.10 | v58.93,32.89 59.18,33.15 59.61,33.15 | 59.61,33.15 U3.8 | 59.61,33.15 arc82 59.23,32.82
  Bottom 0.254: U4.8 54.61,33.78 55.5,32.89 57.91,32.89 | 57.91,32.89 v58.93,32.89 | 57.91,32.89 58.93,33.15 | 57.91,32.89 58.93,32.64
D6  (via drill 0.5 pad 0.9)
  Top 0.203: 18.8,32.51 23.11,32.51 23.75,33.15 27.56,33.15 29.34,33.15 U1.9 40.13,33.15 40.77,33.78 U2.9 56.64,33.78 | 56.64,33.78 56.97,33.78 | 56.97,33.78 57.02,33.78 v57.4,34.16 | 56.97,33.78 arc10 57.53,33.83 | 56.64,33.78 arc93 57.07,34.24
  Top 0.254: 18.8,32.51 18.16,32.51 | v17.4,32.83 18.16,32.51 | v57.4,34.16 57.66,34.42 58.12,34.42 | 58.12,34.42 U3.9 | 18.16,32.51 17.4,32.51 | 18.16,32.51 17.4,33.15 | 58.12,34.42 arc82 57.71,34.06
  Bottom 0.254: CNY.11 14.1,28.32 | 14.1,28.32 14.61,28.32 15.49,29.21 17.4,29.21 18.67,30.48 18.67,31.56 v17.4,32.83 | U4.9 54.74,35.05 55.63,34.16 56.39,34.16 | 56.39,34.16 v57.4,34.16 | 56.39,34.16 57.4,34.42 | 56.39,34.16 57.4,33.91 | 14.1,28.32 12.7,27.69 | 14.1,28.32 12.7,28.96
D7  (via drill 0.5 pad 0.9)
  Top 0.203: 18.8,33.78 22.48,33.78 23.11,34.42 U1.10 38.86,34.42 39.5,35.05 U2.10 55.04,35.05 | 55.04,35.05 55.5,35.05 | 55.5,35.05 v55.88,35.43 | 55.5,35.05 55.52,35.05 arc12 56.01,35.1 | 55.04,35.05 arc87 55.55,35.53
  Top 0.254: 18.8,33.78 17.91,34.67 15.24,34.67 | v55.88,35.43 56.13,35.69 56.62,35.69 | 56.62,35.69 U3.10 | 15.24,34.67 14.61,34.42 | 15.24,34.67 v14.61,34.67 | 56.62,35.69 arc79 56.19,35.33 | 15.24,34.67 14.61,34.92
  Bottom 0.254: 13.72,34.67 9.14,34.67 8.64,34.16 8.64,28.83 8.89,28.58 | 8.89,28.58 9.14,28.32 | 9.14,28.32 CNY.12 | 13.72,34.67 v14.61,34.67 | U4.10 54.99,36.32 55.12,36.2 | 55.12,36.2 v55.88,35.43 | 55.12,36.2 55.88,35.69 | 55.12,36.2 55.63,35.43 | 8.89,28.58 10.16,28.58 | 9.14,28.32 9.4,28.07 10.16,28.07 | 13.72,34.67 14.61,34.92 | 13.72,34.67 14.61,34.42
D8  (via drill 0.5 pad 0.9)
  Top 0.203: U1.33 22.22,34.42 22.86,35.05 U2.33 | 36.96,35.05 U2.33 | U2.33 38.48,35.05 39.12,35.69 U3.33 54.86,35.69 55.5,36.32 65.28,36.32
  Top 0.254: U1.33 19.05,34.42 17.53,35.94 14.1,35.94 | 65.28,36.32 v65.91,36.32 | CNY.17 14.1,35.94 | 14.1,35.94 12.7,36.58 | 14.1,35.94 12.7,35.31
  Bottom 0.254: v65.91,36.32 U4.33
D9  (via drill 0.5 pad 0.9)
  Top 0.203: U1.34 22.73,33.15 23.37,33.78 U2.34 39.5,33.78 40.13,34.42 U3.34 56.26,34.42 56.9,35.05 65.28,35.05
  Top 0.254: CNY.14 11.43,32.13 13.59,32.13 15.24,33.78 17.91,33.78 18.54,33.15 U1.34 | 65.28,35.05 v65.91,35.05
  Bottom 0.254: v65.91,35.05 U4.34
D10  (via drill 0.5 pad 0.9)
  Top 0.203: U1.35 23.49,31.88 24.13,32.51 U2.35 40.77,32.51 41.4,33.15 U3.35 57.78,33.15 58.42,33.78 65.28,33.78
  Top 0.254: U1.35 14.61,31.88 13.84,31.12 | 65.28,33.78 v65.91,33.78 | CNY.13 13.59,30.86 | 13.59,30.86 13.84,31.12 | 13.59,30.86 13.34,30.61 12.7,30.61 | 12.7,31.12 13.84,31.12
  Bottom 0.254: v65.91,33.78 U4.35
D11  (via drill 0.5 pad 0.9)
  Top 0.203: U1.36 24.26,30.61 24.89,31.24 U2.36 42.04,31.24 42.67,31.88 U3.36 59.44,31.88 60.07,32.51 65.28,32.51
  Top 0.254: U1.36 18.41,30.61 | 18.41,30.61 17.91,30.61 | 17.91,30.61 17.4,30.61 v17.27,30.35 | v17.27,30.35 17.91,30.61 | 18.41,30.61 v17.27,30.35 | 65.28,32.51 v65.91,32.51
  Bottom 0.254: CNY.16 11.18,32.38 | 11.18,32.38 11.43,32.13 13.72,32.13 15.49,30.35 v17.27,30.35 | v65.91,32.51 U4.36 | 11.18,32.38 10.03,32.89 | 11.18,32.38 10.67,33.53
D12  (via drill 0.5 pad 0.9)
  Top 0.203: U1.38 22.35,28.07 22.99,28.7 U2.38 41.4,28.7 42.04,29.34 U3.38 56.64,29.34 57.28,29.97 65.28,29.97
  Top 0.254: U1.38 18.67,28.07 | 18.67,28.07 v18.16,28.58 | 18.67,28.07 18.29,28.7 | 18.67,28.07 18.03,28.45 | 65.28,29.97 v65.91,29.97
  Bottom 0.254: v18.16,28.58 19.56,29.97 19.56,32.64 18.03,34.16 16.76,34.16 16,33.4 14.1,33.4 | v65.91,29.97 U4.38 | CNY.15 14.1,33.4 | 14.1,33.4 12.7,32.77 | 14.1,33.4 12.7,34.04
D13  (via drill 0.5 pad 0.9)
  Top 0.203: U1.39 23.62,26.8 24.26,27.43 U2.39 42.42,27.43 43.05,28.07 U3.39 57.91,28.07 58.55,28.7 65.28,28.7
  Top 0.254: U1.39 17.65,26.8 17.4,27.05 | 17.4,27.05 17.27,27.18 | 17.27,27.18 17.14,27.3 | 17.14,27.3 v16.51,27.3 | 17.14,27.3 16.51,27.05 17.4,27.05 | 17.14,27.3 16.51,27.56 | 17.27,27.18 16.51,27.18 | 65.28,28.7 v65.91,28.7
  Bottom 0.254: 15.49,27.05 9.14,27.05 7.87,28.32 7.87,34.67 8.89,35.69 | 15.49,27.05 15.75,27.05 | 8.89,35.69 9.14,35.94 | 9.14,35.94 CNY.18 | v16.51,27.3 15.75,27.05 | 15.75,27.05 16.51,27.05 | 15.49,27.05 16.51,27.56 | v65.91,28.7 U4.39 | 8.89,35.69 10.16,35.69 | 9.14,35.94 9.4,36.2 10.16,36.2
D14  (via drill 0.5 pad 0.9)
  Top 0.203: U1.40 24.89,25.53 25.53,26.16 U2.40 43.43,26.16 44.07,26.8 U3.40 59.31,26.8 59.94,27.43 65.28,27.43
  Top 0.254: U1.40 17.14,25.53 | 17.14,25.53 16.64,25.53 v16.51,25.27 17.14,25.53 | 65.28,27.43 v65.91,27.43
  Bottom 0.254: CNY.19 11.68,37.46 | 11.68,37.46 11.43,37.21 8.89,37.21 7.11,35.43 7.11,26.8 9.4,24.51 15.75,24.51 v16.51,25.27 | v65.91,27.43 U4.40 | 11.68,37.46 12.95,37.97 | 11.68,37.46 12.19,38.73
D15  (via drill 0.5 pad 0.9)
  Top 0.203: 36.96,24.89 U2.41 | U2.41 26.8,24.89 26.16,24.26 U1.41 | U2.41 44.58,24.89 45.21,25.53 U3.41 60.96,25.53 61.59,26.16 65.28,26.16
  Top 0.254: U1.41 18.67,24.26 | 18.67,24.26 18.16,24.26 v18.03,24 18.67,24.26 | 65.28,26.16 v65.91,26.16
  Bottom 0.254: 8.64,38.48 CNY.20 | v18.03,24 16,21.97 9.4,21.97 6.35,25.02 6.35,36.2 8.38,38.23 | U4.41 v65.91,26.16 | 8.38,38.23 8.64,38.48 | 8.38,38.23 10.16,38.23 | 8.64,38.48 8.89,38.73 10.16,38.73
ENABLE  (via drill 0.5 pad 0.9)
  Top 0.203: 65.66,13.72 63.88,14.1 65.66,14.48 | 21.34,13.84 22.86,14.1 21.34,14.35 | EXRAM.1 20.07,56.26
  Top 0.254: SWITCH.1 63.88,14.1 22.86,14.1 v21.34,14.1 | 4.57,21.97 4.83,23.49 5.08,21.97 | 4.57,43.31 4.83,41.78 5.08,43.31
  Top 0.305: v4.83,43.31 4.83,41.78 4.83,23.49 v4.83,21.97
  Bottom 0.254: 11.18,54.74 CNY.32 8.76,53.72 | 11.18,54.74 11.43,54.99 14.48,54.99 15.75,56.26 16.64,56.26 | 8.76,53.72 6.86,53.72 4.83,51.69 v4.83,43.31 | v4.83,21.97 4.83,14.86 7.11,12.57 19.81,12.57 v21.34,14.1 | 8.76,53.72 10.16,53.09 | 8.76,53.72 10.16,54.36 | 11.18,54.74 10.67,53.59 | 11.18,54.74 10.03,54.23 | EXRAM.1 16.64,56.26 | 16.64,56.26 18.03,55.63 | 16.64,56.26 18.03,56.9
GND  (via drill 0.5 pad 0.9, 0.6)  (1 unrouted)
  Top 0.203: 28.96,41.02 v28.83,41.02 | U2.11 | U3.22 53.09,49.66 | 33.02,42.04 33.78,41.53
  Top 0.254: 19.56,50.04 18.67,48.89 18.8,48.77 | U1.42 23.49,22.99 | 18.8,29.34 U1.37 22.35,29.34 | 18.54,36.2 18.8,35.69 U1.32 24.64,35.69 | 49.53,36.7 49.02,37.59 U2.12 45.34,37.59 44.83,37.08 | U2.11 49.66,36.32 49.53,36.45 | U2.32 33.78,36.32 | U1.11 33.91,35.69 33.4,35.94 | 28.96,36.96 U1.12 34.16,36.96 | 34.04,23.62 U2.42 39.5,23.62 | 23.11,49.15 22.35,48.39 19.18,48.39 18.8,48.77 | 34.54,49.02 U2.22 | U2.22 38.86,49.02 39.5,49.66 | 31.11,35.69 28.19,35.69 | U2.22 36.94,50.41 36.2,50.42 | U1.16 33.02,42.04 | U1.15 29.72,40.77 | 29.72,40.77 28.96,41.02 | 33.02,42.04 v33.84,41.78 | U3.32 49.66,36.96 | 53.34,36.96 U3.11 | U3.12 61.72,38.23 61.34,37.85 | 65.53,38.23 65.66,38.1 | U2.16 49.02,42.67 | v50.55,42.42 49.02,42.67 | U2.15 45.85,41.4 | 45.85,41.4 v44.7,41.66 | 62.99,43.31 U3.16 63.75,43.31 | U3.15 63.12,42.04 | 53.21,24.26 U3.42 51.56,24.26 51.56,22.48 | 53.21,24.26 55.37,24.26 55.37,24 | U3.22 53.21,49.66 | 53.21,49.66 54.61,49.66 55.75,50.29 | 53.21,49.66 53.21,50.8 | 53.09,49.66 50.16,49.66 | 29.72,40.77 28.83,40.77 | 45.85,41.4 44.7,41.53 | 49.02,42.67 50.55,42.67 | 49.02,42.67 50.55,42.16 | 33.02,42.04 33.91,42.04 | 45.85,41.4 44.7,41.78 | 45.85,41.4 44.7,41.4 | 22.35,29.34 22.73,29.72 | 36.96,36.32 39.12,36.32 | 46.86,36.32 44.7,36.32 | 20.57,54.23 EXRAM.2 20.57,57.78 | 22.35,29.34 22.94,29.34 23.11,29.52 | 53.21,24.26 53.21,22.61 | 18.8,48.77 18.8,49.02
  Top 0.305: U3.11 66.55,37.34 | U3.12 65.53,38.23 | U3.15 66.55,42.42 | 63.75,43.31 66.55,42.93
  Top 0.406: U1.42 20.69,21.45 20.57,21.34 | U1.22 20.69,49.54 20.57,49.66 | U2.37 38.61,29.97 38.99,29.59 | U3.37 54.86,30.61 55.24,30.35 | U2.42 36.94,22.1 36.96,22.1 | v80.77,31.12 80.77,32.17 IC1.7 | C9.2 81.41,43.18 v80.77,43.81 80.56,44.03 IC2.7 | C17.2 v80.77,55.88 80.56,56.1 IC3.7 | C18.2 v80.77,68.58 80.56,68.8 IC4.7 | C24.2 v80.77,81.28
  Top 0.508: v40.89,29.59 v39.62,29.59 38.99,29.59 | 55.24,30.35 v56.26,30.35
  Top 0.61: SOCKET(MOBO).24 GARY.24 | SOCKET(MOBO).1 GARY.1
  Bottom 0.203: 63.37,31.37 62.23,31.37
  Bottom 0.254: U4.11 50.93,37.59 | 52.96,43.94 52.95,43.93 53.19,43.93 U4.16 | 50.55,43.81 50.67,43.94 U4.16 | U4.32 65.91,37.59 | 63.12,37.59 60.83,37.59 | 51.18,38.86 U4.12 55.24,38.86 | 53.21,37.59 55.5,37.59 | 50.8,42.67 U4.15 55.75,42.67 | 63.63,51.56 63.88,51.82 | 63.63,24.89 U4.42 66.29,24.89 | 63.63,24.89 63.63,23.62 | 63.63,24.89 61.09,24.89 | 55.23,43.94 U4.16
  Bottom 0.305: U4.22 66.17,50.29 | 63.63,50.29 63.63,51.56 | 65.02,31.24 62.36,31.24 62.23,31.37 60.83,32.77
  Bottom 0.356: U4.37 65.02,31.24 65.79,31.24
  Bottom 0.406: GARY.1 77.6,84.45
  Bottom 0.61: SOCKET(MOBO).1 GARY.1 | GARY.40 SOCKET(MOBO).40 | SOCKET(MOBO).24 GARY.24
  other vias: 17.91,37.59 37.21,20.19 39.75,20.19 22.86,29.72 52.7,20.32 53.98,20.32 55.24,20.32 43.31,37.21 6.35,70.23 6.35,67.69 52.58,58.67 50.55,83.95 38.48,20.19 53.72,58.67
  pour Top (isolate 0.305): 0.51,88.77 67.69,88.77 67.69,0.13 0.51,0.13
  pour Bottom (isolate 0.305): 0.64,88.77 67.44,88.77 67.44,0.63 0.64,0.63
  pour Top: 9.02,30.73 19.68,30.73 19.68,24.51 9.02,24.51
  pour Top: 14.35,40 55.63,40 55.88,34.54 14.35,34.54
  pour Bottom (isolate 0.305): 77.6,24.89 77.6,85.6 89.03,85.6 89.03,24.89
N$1
  Bottom 0.254: R6.P$1 LED.P$2
N$2
  Top 0.305: SOCKET(MOBO).47 GARY.47
N$3
  Top 0.305: SOCKET(MOBO).46 GARY.46
N$4
  Top 0.305: SOCKET(MOBO).45 GARY.45
N$5  (via drill 0.6)
  Top 0.254: IC1.3 v81.79,37.46 | v79.76,84.2 85.34,84.2 87.12,85.98 JP9.1 85.19,87.38
  Bottom 0.254: v79.76,84.2 79.76,51.69 82.8,48.64 84.96,48.64 85.73,47.88 85.73,43.94 81.79,40 v81.79,37.46
N$6
  Top 0.305: GARY.43 SOCKET(MOBO).43
N$7
  Bottom 0.305: GARY.42 SOCKET(MOBO).42
N$11
  Top 0.406: 45.83,76.96 R5.P$2
  Top 0.61: R5.P$2 46.21,69.24 BAT1.+
N$12
  Top 0.406: D1.2 44.05,78.7 R4.P$1
N$14
  Top 0.305: SOCKET(MOBO).44 GARY.44
N$15
  Bottom 0.305: GARY.34 SOCKET(MOBO).34
N$16
  Top 0.406: D1.1 44.3,77 R5.P$1
N$17
  Bottom 0.305: GARY.32 SOCKET(MOBO).32
N$18
  Bottom 0.305: GARY.31 SOCKET(MOBO).31
N$19
  Bottom 0.305: GARY.30 SOCKET(MOBO).30
N$20
  Bottom 0.305: GARY.29 SOCKET(MOBO).29
N$21
  Bottom 0.305: GARY.28 SOCKET(MOBO).28
N$23
  Bottom 0.305: GARY.26 SOCKET(MOBO).26
N$24
  Bottom 0.305: GARY.25 SOCKET(MOBO).25
N$25  (via drill 0.6)
  Top 0.254: v84.58,66.67 84.58,64.14 83.31,62.86 83.31,60.96 82.04,59.69 IC3.6
  Top 0.305: IC4.2 v83.95,77.47
  Bottom 0.305: v83.95,77.47 84.58,76.84 v84.58,66.67
N$26
  Top 0.305: IC3.9 IC3.10 IC3.11
N$27  (via drill 0.6)
  Top 0.254: IC3.3 82.68,63.5 83.31,64.14 v83.31,65.41
  Top 0.305: v83.31,76.2 IC4.12
  Bottom 0.305: v83.31,65.41 v83.31,76.2
N$28  (via drill 0.6)
  Top 0.305: IC1.1 79.92,40.64 v79.5,40.64
  Bottom 0.254: v79.5,40.64 78.87,40 78.87,28.19 77.98,27.3 75.95,27.3
  Bottom 0.305: 75.95,27.3 73.15,27.3 72.64,26.8 72.64,24.77 73.15,24.26 74.93,24.26 JP8.2
N$29  (via drill 0.6)
  Top 0.254: v87.76,67.95 87.25,67.44 87.25,51.56 86.49,50.8
  Top 0.305: 86.49,50.8 IC2.12 v84.58,50.8 | v84.58,34.92 IC1.10 IC1.9
  Bottom 0.254: JP9.2 84.58,86.23 85.34,85.47 86.74,85.47 87.76,84.45
  Bottom 0.305: v84.58,50.8 85.98,50.8 87.25,49.53 87.25,36.2 85.98,34.92 v84.58,34.92 | 87.76,84.45 v87.76,67.95
N$30
  Top 0.254: 86.49,37.46 87.25,36.7 87.25,33.15 86.49,32.38
  Top 0.305: IC1.12 86.49,37.46 | 86.49,32.38 IC1.8
N$31  (via drill 0.6)
  Top 0.305: IC2.13 v83.95,52.07 | v82.68,33.66 IC1.6 | IC1.13 v84.58,38.73
  Bottom 0.305: v83.95,52.07 85.98,52.07 87.88,50.16 87.88,34.92 86.61,33.66 v82.68,33.66 82.68,34.8 84.58,36.7 v84.58,38.73
OE  (via drill 0.5 pad 0.9)
  Top 0.203: 25.53,39.5 26.42,40.39 27.56,40.39 27.81,40.13 U2.29 38.61,40.13 39.24,40.77 U3.29 | 61.98,41.4 65.28,41.4
  Top 0.254: 25.53,39.5 U1.29 14.1,39.5 13.84,39.75 8.89,39.75 6.99,41.66 6.99,54.36 8.89,56.26 CNY.34 | U3.29 56.64,40.77 57.28,41.4 61.98,41.4 | 65.28,41.4 v65.91,41.4
  Bottom 0.254: v65.91,41.4 U4.29
ORIGA19  (via drill 0.6)
  Top 0.305: v83.31,53.34 IC2.1 IC2.2
  Bottom 0.254: JP2.1 75.69,18.41 77.72,18.41 78.23,18.92 78.23,20.95 JP8.1
  Bottom 0.305: v83.31,53.34 87.25,53.34 SOCKET(MOBO).35 GARY.35 93.6,50.04 93.6,24.89 91.95,23.24 85.09,23.24 82.42,25.91 80.65,25.91 79.5,24.77 JP8.1
ORIGA20  (via drill 0.6)
  Top 0.254: v85.22,26.67 85.22,30.48 84.07,31.62 84.07,33.91 82.8,35.18 82.8,38.23 82.3,38.73 82.04,38.73 | SOCKET(MOBO).36 90.4,52.73 90.4,24.99 90.17,24.77 v87.12,24.77
  Top 0.305: v85.22,26.67 82.17,23.62 80.65,23.62 80.39,23.88 74.93,23.88 74.42,23.37 JP8.3 JP6.1 | IC1.2 82.04,38.73
  Bottom 0.305: GARY.36 SOCKET(MOBO).36 | v87.12,24.77 v85.22,26.67
ORIGN$5
  Bottom 0.305: GARY.41 SOCKET(MOBO).41
ORIGN$9
  Bottom 0.305: GARY.38 SOCKET(MOBO).38
ORIGN$10
  Bottom 0.305: GARY.37 SOCKET(MOBO).37
ORIGN$13
  Bottom 0.305: GARY.33 SOCKET(MOBO).33
ORIGN$22
  Top 0.254: IC2.8 85.22,45.72 84.58,45.09 83.31,45.09 82.68,45.72 82.68,46.99 81.41,48.26 IC2.5
P2
  Top 0.305: SOCKET(MOBO).2 GARY.2
P3
  Top 0.305: SOCKET(MOBO).3 GARY.3
P4
  Top 0.305: SOCKET(MOBO).4 GARY.4
P5
  Top 0.305: SOCKET(MOBO).5 GARY.5
P7
  Top 0.305: GARY.7 SOCKET(MOBO).7
P8
  Top 0.305: GARY.8 SOCKET(MOBO).8
P9
  Top 0.305: GARY.9 SOCKET(MOBO).9
P10
  Top 0.305: GARY.10 SOCKET(MOBO).10
P11
  Top 0.305: GARY.11 SOCKET(MOBO).11
P12
  Top 0.305: GARY.12 SOCKET(MOBO).12
P13
  Top 0.305: GARY.13 SOCKET(MOBO).13
P14
  Top 0.305: GARY.14 SOCKET(MOBO).14
P16
  Bottom 0.305: GARY.16 SOCKET(MOBO).16
P19
  Bottom 0.305: GARY.19 SOCKET(MOBO).19
P21
  Top 0.305: GARY.21 SOCKET(MOBO).21
P22
  Top 0.305: GARY.22 SOCKET(MOBO).22
P23
  Top 0.305: GARY.23 SOCKET(MOBO).23
RAS0  (via drill 0.5 pad 0.9)
  Top 0.254: v55.12,56.26 v38.61,56.26 26.92,56.26 23.37,52.7 JP1.1
  Bottom 0.254: JP1.1 23.37,59.56 21.59,61.34 14.1,61.34 | CNY.37 14.1,61.34 | JP5.1 v55.12,56.26 55.12,59.94 54.23,60.83 SJ1.1 | JP7.1 39.62,55.24 v38.61,56.26 | 14.1,61.34 12.7,61.98 | 14.1,61.34 12.7,60.71
RAS1
  Top 0.254: JP7.3 44.7,54.74 | 26.42,51.18 JP1.3 28.45,52.7 30.48,54.74 44.7,54.74 | 44.7,54.74 59.05,54.74 60.2,53.59 JP5.3 58.42,52.45
  Bottom 0.254: CNY.38 11.18,62.36 | 11.18,62.36 11.43,62.61 22.86,62.61 28.45,57.02 JP1.3 | 51.13,60.83 SJ1.3 50.16,62.23 50.93,62.99 56.01,62.99 60.2,58.8 JP5.3 | 11.18,62.36 10.67,61.09 | 11.18,62.36 9.91,61.85
RAS_CTL
  Top 0.254: J8.1 85.85,20.45 85.85,25.4 87.88,27.43 87.88,41.78 85.22,44.45 82.68,44.45 82.04,45.09 82.04,46.35 81.41,46.99 IC2.6
RASU1  (via drill 0.5 pad 0.9)
  Top 0.203: 26.8,39.24 27.94,39.5 26.8,39.75
  Top 0.254: U1.14 27.94,39.5 v26.8,39.5
  Bottom 0.254: JP1.2 25.91,42.8 25.15,42.04 25.15,40.77 26.16,39.75 26.29,39.62 | 26.29,39.62 26.42,39.5 v26.8,39.5 | 26.29,39.62 26.8,39.62 | 26.29,39.62 26.67,39.24
RASU2  (via drill 0.5 pad 0.9)
  Top 0.254: U2.14 42.55,40.13 | 42.55,40.13 v41.15,39.5 | 42.55,40.13 41.15,39.24 | 42.55,40.13 41.15,39.75
  Bottom 0.254: JP7.2 42.16,40.51 v41.15,39.5
RASU3  (via drill 0.5 pad 0.9)
  Top 0.254: U3.14 61.21,40.77 60.71,40.26 59.31,40.26 | 59.31,40.26 v58.17,40.26 | 59.31,40.26 58.17,40 | 59.31,40.26 58.17,40.51
  Bottom 0.254: JP5.2 57.66,47.88 59.18,46.35 59.18,44.96 58.17,43.94 58.17,41.27 | v58.17,40.26 58.17,41.27 | 58.17,41.27 58.42,40.26 | 58.17,41.27 57.91,40.26
RASU4
  Bottom 0.254: U4.14 50.29,41.4 49.53,42.16 49.53,49.53 51.31,51.31 51.31,60.2 SJ1.2
  Bottom 0.406: 53.21,41.4 U4.14
SEL0
  Bottom 0.305: JP2.2 78.49,15.62 83.31,15.62 84.07,16.38 84.07,18.16 J8.2
SEL1
  Top 0.254: JP6.2 78.23,20.95 81.28,20.95 J8.3
STD.P
  Top 0.254: R2.P$1 42.42,84.96 41.66,85.73 37.08,85.73 U5.1 36.2,84.84 | 36.2,84.84 36.83,84.84 | 36.2,84.84 36.2,85.47 | U55.1 34.43,83.07 36.2,84.84
VBAT
  Top 0.254: 39.62,77.85 D1.3
  Top 0.406: 39.62,77.85 U5.18 36.83,75.33 C12.P$2 34.54,75.31 33.66,74.42 U55.24
  Bottom 0.254: 39.62,77.85 C19.P$1
  Bottom 0.406: C13.P$1 U5.18 39.62,77.85
VCC  (via drill 0.5 pad 0.9, 0.6 pad 1.22, 0.7 pad 1.27)  (2 unrouted)
  Top 0.254: 84.31,73.66 84.31,73.93 83.95,74.3 82.04,74.3 81.41,74.93 IC4.4 79.38,74.93 | 77.6,71.75 79.38,73.53 79.38,74.93 | 79.38,74.93 79.38,77.98 80.14,78.74 | C9.1 84.31,42.27 83.95,41.91 81.28,41.91 79.38,43.81 GARY.17
  Top 0.305: IC2.14 86.07,55.03 85.22,55.88 C17.1 84.31,62.59 85.22,63.5 IC3.12 IC3.13 IC3.14 86.07,67.73 85.22,68.58 C18.1 84.31,73.66 IC4.10 | SOCKET(MOBO).48 87.76,83.06 87.76,80.01 86.49,78.74 IC4.14 | C24.1 85.22,81.28 86.07,80.43 IC4.14 | GARY.6 77.6,71.75 | 80.14,78.74 IC4.1 IC4.14 | IC4.13 IC4.14 | IC1.14 86.07,42.33 85.22,43.18 C9.1
  Top 0.406: U1.6 29.46,29.34 29.08,29.72 | 31.11,48.39 U1.21 32.77,48.39 33.13,48.75 C2.P$2 33.13,52.69 33.4,52.96 v34.29,52.96 | U2.6 45.97,29.97 45.72,30.23 | 63.87,49.66 U3.21 | U6.16 v57.91,86.87 | 63.25,49.66 U3.21 | U3.6 62.23,30.61 | 62.23,30.61 v61.21,30.86 | v47.88,53.09 49.4,53.09 | 49.4,53.09 v52.58,53.09 | 62.23,30.61 61.21,30.61 | U1.1 31.1,22.99 | 31.11,20.57 31.11,20.45 C1.P$2 | U2.1 47.35,23.62 | U2.21 49.02,49.02 49.39,49.39 C5.P$2 49.39,53.07 49.4,53.09 | C8.P$2 64.91,50.05 64.52,49.66 U3.21
  Top 0.508: 29.08,29.72 v28.32,29.72 v27.05,29.72 | v43.81,30.23 v45.09,30.23 45.72,30.23
  Top 0.61: CNY2.12 CNY2.11 14.22,79.12 15.49,80.39 35.31,80.39 36.85,81.93 R1.P$2 | 39.86,81.66 R1.P$2 | R1.P$2 R2.P$2 R3.P$2 R7.P$1 47.5,80.9 v48.01,80.39 48.01,79.12 | 65.79,56.77 66.22,56.34 C20.+ 66.22,54.79 64.91,53.48 C8.P$2 | 65.79,56.77 48.01,74.55 48.01,79.12 | U3.1 63.64,21.72 C7.P$2 63.63,21.72 63.63,17.91 | R4.P$2 48.01,79.12 | GARY.48 SOCKET(MOBO).48 | GARY.6 SOCKET(MOBO).6 | SOCKET(MOBO).17 GARY.17 | 31.1,22.99 C1.P$2 | 31.11,20.45 31.11,17.91 | 47.35,23.62 C4.P$2 47.37,21.08 47.37,17.91 | 65.79,56.77 65.79,56.01
  Top 1.219: CNY.2 CNY.1 17.27,15.62 19.56,17.91 31.11,17.91 47.37,17.91 63.63,17.91
  Bottom 0.254: 48.01,82.68 v48.01,80.39
  Bottom 0.305: 48.01,82.68 48.01,83.69 51.69,87.38 51.82,87.38 v57.91,86.87 57.91,84.98 C16.P$1 | SOCKET(MOBO).17 72.52,45.21 72.52,70.36 SOCKET(MOBO).6
  Bottom 0.406: 51.05,29.59 51.05,30.86 51.44,31.24 U4.6 54.99,31.24 55.37,31.62 60.45,31.62 v61.21,30.86 | 51.05,29.59 51.05,29.08 | U4.21 52.58,50.29 | C21.P$2 52.58,55.39 | R6.P$2 33.02,24.77 32.89,24.89 | 50.8,29.34 51.05,29.08 | 50.8,29.34 51.05,29.59 | 46.23,24.89 46.23,23.37 47.37,22.23 C22.P$2 52.98,24.67 U4.1 | 51.05,29.08 51.05,27.56 48.77,25.27 | 48.01,24.89 48.39,24.89 48.77,25.27 | 50.8,29.34 48.12,29.34 C23.P$2 | C11.P$1 48.01,80.44 v48.01,80.39 | 48.77,25.27 47.75,25.27
  Bottom 0.61: v27.05,29.72 v28.32,29.72 | v43.81,30.23 v45.09,30.23 | v34.29,52.96 34.29,47.12 35.81,45.59 35.81,25.15 36.07,24.89 | 28.32,24.89 v28.32,29.72 | v47.88,53.09 46.23,51.43 46.23,30.23 | v43.81,30.23 46.23,30.23 | v43.81,30.23 43.81,31.99 C6.P$2 | 46.23,30.23 46.23,24.89 | 52.58,50.29 v52.58,53.09 52.58,55.39 | SOCKET(MOBO).48 GARY.48 | SOCKET(MOBO).6 GARY.6 | C3.P$2 28.32,32 v28.32,29.72
  Bottom 1.219: CNY.2 CNY.1 17.27,15.62 26.54,24.89 28.32,24.89 32.89,24.89 36.07,24.89 46.23,24.89 48.01,24.89
WE  (via drill 0.5 pad 0.9)
  Top 0.203: U1.13 41.66,38.23 42.29,38.86 U2.13 55.63,38.86 | 29.34,38.23 28.07,37.72
  Top 0.254: U1.13 29.34,38.23 | 56.13,38.86 55.63,38.86 55.88,39.12 56.13,38.86 | 56.13,38.86 60.96,38.86 61.59,39.5 U3.13 | CNY.39 11.43,62.61 9.02,62.61 8.51,62.1 8.51,58.04 9.02,57.53 14.99,57.53 15.88,56.64 15.88,53.72 16.76,52.83 v20.83,52.83 | 29.34,38.23 v27.94,37.97 | 29.34,38.23 27.94,38.23
  Top 0.406: v55.88,39.75 55.88,39.12
  Bottom 0.254: v20.83,52.83 20.83,43.31 26.16,37.97 v27.94,37.97 | U4.13 55.24,40.13 | 55.24,40.13 55.5,40.13 | 55.5,40.13 v55.88,39.75 | 55.5,40.13 55.88,40.13 56.13,39.88 | 55.24,40.13 55.88,39.5
XA2
  Top 0.254: U55.5 28.57,84.84 | 28.57,84.84 U5.4 | 28.57,84.84 29.21,84.84 | 28.57,84.84 28.57,85.47
  Bottom 0.254: U5.4 29.21,82.93 25.91,79.63 18.54,79.63 17.78,78.87 17.78,75.56 13.97,71.75 | CNY2.5 13.72,71.5 | 13.97,71.75 13.72,71.5 | 13.97,71.75 12.7,71.75 | 13.72,71.5 13.46,71.25 12.7,71.25
XA3
  Top 0.254: U55.7 26.04,84.84 | 26.04,84.84 U5.5 | 26.04,84.84 26.67,84.84 | 26.04,84.84 26.04,85.47
  Bottom 0.254: U5.5 26.67,82.68 25.15,81.15 16.51,81.15 14.22,78.87 14.22,75.82 13.72,75.31 11.94,75.31 11.43,74.8 11.43,72.77 CNY2.6
XA4
  Top 0.254: CNY2.7 11.43,72.77 9.4,72.77 7.37,74.8 7.37,85.22 10.03,87.88 21.72,87.88 U5.6 23.49,84.84 | U55.9 23.49,84.84 | 23.49,84.84 24.13,84.84 | 23.49,84.84 23.49,85.47
XA5
  Top 0.254: CNY2.8 8.13,76.07 8.13,84.71 10.54,87.12 19.94,87.12 U5.7 22.22,84.84 | U55.10 22.22,84.84 | 22.22,84.84 21.59,84.84 | 22.22,84.84 22.22,85.47
XCASL  (via drill 0.5 pad 0.9)
  Top 0.254: 13.21,58.8 CNY.35 14.1,58.8 | JP10.3 33.53,63.88 | JP10.7 28.45,65.66 | 28.45,65.66 28.45,63.88 | JP10.7 27.43,65.91 | 27.43,65.91 27.18,65.66 | 27.18,65.66 26.92,65.41 | JP10.7 27.18,65.66 | 27.18,65.66 28.45,65.66 | 27.43,65.91 27.94,66.42 | 26.92,65.41 28.19,65.41 | U6.1 52.58,86.87 52.2,86.49 v52.2,85.73 | 14.1,58.8 12.7,58.17 | 14.1,58.8 12.7,59.44 | 26.92,65.41 25.53,64.01 25.4,63.88 25.15,63.63 16.51,63.63 16,63.12 16,60.58 14.22,58.8 14.1,58.8
  Bottom 0.254: JP10.7 29.84,67.31 32.13,67.31 JP10.3 33.53,67.82 37.08,71.37 46.23,71.37 53.98,79.12 53.98,83.95 v52.2,85.73
XCASU  (via drill 0.5 pad 0.9)
  Top 0.254: CNY.36 11.43,60.07 13.97,60.07 14.99,61.09 14.99,63.88 15.75,64.64 24.38,64.64 27.05,67.31 30.61,67.31 | 36.07,63.88 JP10.1 35.05,66.93 34.67,67.31 31.37,67.31 | 30.99,63.88 JP10.5 30.99,67.31 | U6.15 v62.36,85.6 | 30.61,67.31 30.73,67.31 | 30.73,67.31 30.99,67.31 | 30.99,67.31 31.24,67.31 | 31.24,67.31 31.37,67.31 | 30.73,67.31 30.73,67.18 | 30.73,67.18 30.73,66.42 | 31.24,67.31 31.24,67.18 | 31.24,67.18 31.24,66.42 | 30.61,67.31 30.73,67.18 | 31.37,67.31 31.24,67.18
  Top 0.305: 35.56,65.79 35.05,66.93 36.2,66.42
  Bottom 0.254: JP10.1 36.07,67.56 38.1,69.6 47.24,69.6 57.15,79.5 57.15,81.15 61.59,85.6 v62.36,85.6
XCLKCS
  Top 0.203: CLOCK.2 18.67,59.18
  Bottom 0.254: CLOCK.2 19.18,57.78 15.75,57.78 14.35,56.39 | CNY.33 14.1,56.26 | 14.1,56.26 14.22,56.26 | 14.22,56.26 14.35,56.39 | 14.1,56.26 12.7,55.63 | 14.1,56.26 12.7,56.9 | 14.22,56.26 14.1,56.13 12.7,56.13 | 14.35,56.39 12.7,56.39
XCLKRD
  Top 0.254: U5.8 19.43,85.47 19.81,85.09 | 19.81,85.09 20.83,84.07 20.83,83.26 U55.11 | 19.81,85.09 19.68,85.09 | 19.68,85.09 19.05,85.09 | 19.68,85.09 19.68,85.47
  Bottom 0.254: CNY2.9 11.43,77.85 11.43,85.22 11.94,85.73 13.72,85.73 15.75,83.69 17.27,83.69 U5.8
XCLKWR
  Top 0.254: U55.13 19.68,74.68 U5.10 13.97,75.31 11.43,75.31 CNY2.10
XD0
  Top 0.254: U55.19 27.3,75.44 26.67,76.07 U5.14
  Bottom 0.254: CNY2.1 14.1,66.42 | 14.1,66.42 14.48,66.42 | 14.48,66.42 14.61,66.55 | 14.61,66.55 23.37,75.31 24.13,75.31 U5.14 | 14.1,66.42 12.7,67.06 | 14.1,66.42 12.7,65.79 | 14.48,66.42 14.35,66.29 12.7,66.29 | 14.61,66.55 12.7,66.55
XD1
  Top 0.254: U55.16 23.49,75.44 24.13,76.07 U5.13
  Bottom 0.254: CNY2.2 11.43,67.69 14.22,67.69 24.13,77.6 U5.13
XD2
  Top 0.254: U55.15 22.22,75.44 21.59,76.07 U5.12
  Bottom 0.254: U5.12 21.59,76.58 14.22,69.22 | 14.22,69.22 13.97,68.96 | 13.97,68.96 CNY2.3 | 14.22,69.22 12.7,69.22 | 13.97,68.96 13.72,68.71 12.7,68.71
XD3
  Top 0.254: U55.14 20.95,74.8 19.05,76.71 U5.11
  Bottom 0.254: CNY2.4 11.43,70.23 13.72,70.23 19.05,75.56 U5.11
XT1
  Top 0.254: U5.17 34.29,76.58 32.38,74.68 U55.23 32.38,71.5 32.26,71.37 | 32.26,71.37 29.97,69.09 25.91,69.09 23.49,66.67 JP3.1 22.87,66.67 Y1.4 | 32.26,71.37 32.26,71.63
  Bottom 0.406: JP3.1 C14.P$1
XT2
  Top 0.254: U5.16 31.75,76.07 31.11,75.44 U55.22 31.11,71.5 30.99,71.37 | 30.99,71.37 29.59,69.98 JP4.1 22.87,69.98 Y1.1 | 30.99,71.37 30.99,71.63
  Bottom 0.406: JP4.1 C15.P$1

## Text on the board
Bottom: PZ
tPlace: 1 | 48 | SEL0 | 56 | 74F139 | REAL TIME CLOCK | MSM6242B | SEL1 | RTC62423 | MC306 | XCAS | CR2032 | CUT THESE FOR / GARY ADAPTER | CAS1L | CAS1U | CAS2L | CAS2U | ENABLE | RAS0 | RASU1 | RAS1 | RAS0 | RASU2 | RAS1 | RAS1 | RAS0 | RASU3 | SOJ42 / 1Mx16 DRAM | SEL1 | 42 | JP3 | TO / TRAP / DOOR | SEL0 | JP1&2 | RASC | TO / MID / JP2 | A500 Trapdoor Memory Expansion / REV B.5 (2017/9/17)
bPlace: Original design: PeteAU / Additional logic: Mathesar / Additional artwork: Mq666 | 56 | 55 | RAS1 | RASU4 | RAS0 | 40 | 39 | THIS ADAPTER / FUDGES RAMEN / AND REGEN FOR / 1.5MB RAM AT $C0 | DISABLE FOR / CHIP RAM: | JP2 wire not / needed for / half meg chip | SEL1 | TO / TRAP / DOOR | SEL0 | RASC | TO / MID / JP2 | 2 | 1 | Configurations: / - A500: 0.5 MB / - A500+: 1.0 MB / - GARY adapter: 2.0 MB
tNames: 512K | JP4 | MORE | GARY / ADAPTER | SLOW | CHIP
